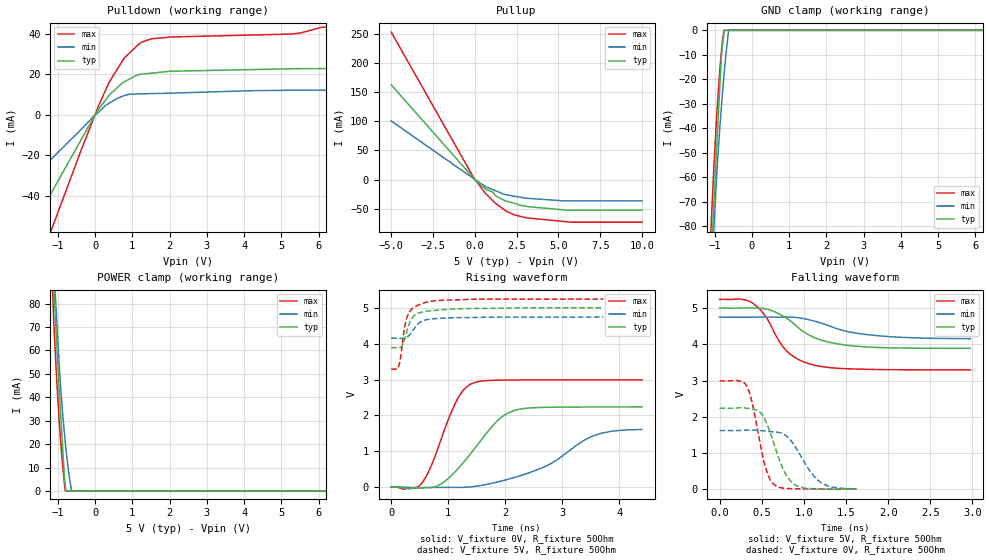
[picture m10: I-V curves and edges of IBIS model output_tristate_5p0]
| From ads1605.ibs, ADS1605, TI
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|   OUTPUT 5.0V Model
[Model]   output_tristate_5p0
Model_type   3-state
Polarity   Non-Inverting
Enable   Active-Low
Vmeas = 1.65
Vref = 1.65
Cref = 15pF
Rref = 50
|   typ   min   max
|   (nom PVT)   (Fast PVT)   (Slow PVT)
|Average
C_comp   2.110e-12   1.917e-12   2.343e-12
|ON state : BUFFER OUTPUT TURNED HIGH
|C_comp   2.191e-12   2.447e-12   2.011e-12
|OFF state: BUFFER in HIGH IMPEDANCE for IOs and 3-state
|C_comp   2.029e-12   2.240e-12   1.824e-12
|Where nom PVT is NOM Process, 3.3V,39C
|   Fast PVT is Strong Process, 3.6V, -40C
|   Slow PVT is Weak Process, 3.0V, 99C
[Voltage Range]   5   4.75   5.25
|Ambient Temperature   25   85   -40
|Junction Temperature
[Temperature Range]   39   99   -40
[Pullup Reference]   5   4.75   5.25
[Pulldown Reference]   0   0   0
[Power Clamp Reference]   5   4.75   5.25
[GND Clamp Reference]   0   0   0
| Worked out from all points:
|   slope of the pulldown table from 0 to 0.75 V, typ, clamps not added: 46.8 ohm
|   slope of the pullup table from 0 to 0.75 V, typ, clamps not added: 42.6 ohm
|   GND clamp passes 1 mA (typ) near -0.74 V on its own axis
|   POWER clamp passes 1 mA (typ) near -0.79 V on its own axis
|   falling waveform, V_fixture 5V, R_fixture 50Ohm: 20-80 % time 460ps typ, 589ps min, 344ps max; typ from 5 V to 3.89 V
|   rising waveform, V_fixture 0V, R_fixture 50Ohm: 20-80 % time 692ps typ, 1.1ns min, 438ps max; typ from 0 V to 2.24 V
|   rising waveform, V_fixture 5V, R_fixture 50Ohm: 20-80 % time 166ps typ, 205ps min, 138ps max; typ from 3.89 V to 5 V
|   falling waveform, V_fixture 0V, R_fixture 50Ohm: 20-80 % time 211ps typ, 270ps min, 160ps max; typ from 2.24 V to 0.006 V
[Pulldown]
|   Voltage   I(typ)   I(min)   I(max)
-5V       -164.5mA   -91.48mA   -246.1mA
-385mV    -12.67mA   -7.415mA   -18.05mA
85mV      2.502mA    1.123mA    4.078mA
381.2mV   9.787mA    5.817mA    16.24mA
785.5mV   16.39mA    9.582mA    28.19mA
1.105V    19.53mA    10.35mA    33.77mA
1.258V    20.16mA    10.42mA    36.01mA
1.505V    20.63mA    10.54mA    37.62mA
2.035V    21.61mA    10.77mA    38.52mA
5.253V    22.81mA    12.22mA    39.98mA
6.104V    22.9mA     12.24mA    43.44mA
10V       22.9mA     12.24mA    43.44mA
[GND Clamp]
|   Voltage   I(typ)   I(min)   I(max)
-5V       -1.587A    -1.343A    -1.956A
-1.089V   -94.33mA   -101.7mA   -79.17mA
-1.02V    -71.99mA   -81.86mA   -57.02mA
-1.01V    -68.66mA   -78.82mA   -53.87mA
-934mV    -45.4mA    -57.09mA   -33.41mA
-868.2mV  -26.14mA   -42.25mA   -18.4mA
-815mV    -10.83mA   -31.39mA   -8.578mA
-779mV    -5.271mA   -24.29mA   -3.416mA
-740mV    -524.8uA   -17.51mA   0A
-696.5mV  0A         -10.25mA   0A
-620.5mV  0A         0A         0A
10V       0A         0A         0A
[Pullup]
|   Voltage   I(typ)   I(min)   I(max)
-5V       163.1mA    100.8mA    253.8mA
0V        0A         0A         0A
620mV     -15.93mA   -12.21mA   -23.08mA
1.11V     -22.2mA    -17.72mA   -37.42mA
1.237V    -28.19mA   -19.16mA   -41.13mA
1.731V    -35.37mA   -25.44mA   -51.39mA
1.914V    -37.55mA   -26.41mA   -55.16mA
2.424V    -41.28mA   -29.04mA   -61.51mA
3.153V    -46.62mA   -32.41mA   -66.25mA
5.804V    -52.76mA   -36.71mA   -73.51mA
10V       -52.76mA   -36.71mA   -73.51mA
[POWER Clamp]
|   Voltage   I(typ)   I(min)   I(max)
-5V       1.555A     1.324A     1.885A
-1.148V   101.3mA    107.1mA    90.18mA
-1.115V   89.74mA    97.82mA    75.94mA
-1.094V   83.11mA    91.87mA    67.95mA
-1.07V    75.59mA    85.06mA    60.54mA
-1.031V   64.07mA    74.01mA    48.52mA
-947mV    39.62mA    50.19mA    26.8mA
-815mV    4.856mA    23.73mA    2.438mA
-794.7mV  2.08mA     20.28mA    0A
-710.7mV  0A         8.426mA    0A
-625.2mV  0A         0A         0A
10V       0A         0A         0A
[Ramp]
R_load = 50
|   typ   min   max
dV/dt_r   1.34161/6.91503e-10   0.971156/1.09954e-09   1.79262/4.38461e-10
dV/dt_f   0.666068/4.61225e-10   0.359082/6.03059e-10   1.169/3.44688e-10
[Falling Waveform]
V_fixture = 5V
V_fixture_min = 4.75V
V_fixture_max = 5.25V
R_fixture = 50Ohm
|   Time   V(typ)   V(min)   V(max)
0s        5V         4.75V      5.242V
250ps     5.002V     4.749V     5.248V
400ps     5.005V     4.751V     5.125V
550ps     4.977V     4.755V     4.758V
700ps     4.848V     4.754V     4.114V
800ps     4.712V     4.756V     3.808V
1.075ns   4.242V     4.672V     3.457V
1.35ns    4.036V     4.469V     3.351V
1.75ns    3.929V     4.27V      3.313V
2.975ns   3.891V     4.157V     3.295V
[Rising Waveform]
V_fixture = 0V
V_fixture_min = 0V
V_fixture_max = 0V
R_fixture = 50Ohm
|   Time   V(typ)   V(min)   V(max)
0s        1.037nV    1.47nV     3.661mV
550ps     -12.88mV   -15.95mV   137.1mV
825ps     46.55mV    -5.923mV   1.105V
1.125ns   433.8mV    -6.267mV   2.338V
1.425ns   997.9mV    13.44mV    2.892V
1.875ns   1.868V     147.6mV    2.982V
2.2ns     2.155V     287.9mV    2.987V
2.775ns   2.227V     635mV      2.99V
3.575ns   2.234V     1.448V     2.991V
4.4ns     2.236V     1.609V     2.991V
[Rising Waveform]
V_fixture = 5V
V_fixture_min = 4.75V
V_fixture_max = 5.25V
R_fixture = 50Ohm
|   Time   V(typ)   V(min)   V(max)
0s        3.89V      4.151V     3.294V
125ps     3.883V     4.152V     3.333V
150ps     3.885V     4.149V     3.474V
200ps     3.965V     4.144V     4.049V
250ps     4.194V     4.156V     4.574V
300ps     4.48V      4.207V     4.827V
400ps     4.777V     4.412V     5.011V
575ps     4.891V     4.648V     5.136V
1.475ns   4.98V      4.731V     5.238V
3.725ns   5V         4.745V     5.242V
[Falling Waveform]
V_fixture = 0V
V_fixture_min = 0V
V_fixture_max = 0V
R_fixture = 50Ohm
|   Time   V(typ)   V(min)   V(max)
0s        2.236V     1.623V     2.991V
250ps     2.252V     1.625V     2.986V
325ps     2.238V     1.633V     2.843V
400ps     2.211V     1.636V     2.249V
550ps     1.874V     1.606V     562.8mV
650ps     1.225V     1.585V     128.1mV
775ps     456.2mV    1.502V     29.58mV
900ps     116.4mV    1.167V     18.2mV
1.2ns     12.84mV    192mV      10.15mV
1.625ns   5.528mV    15.11mV    6.731mV
